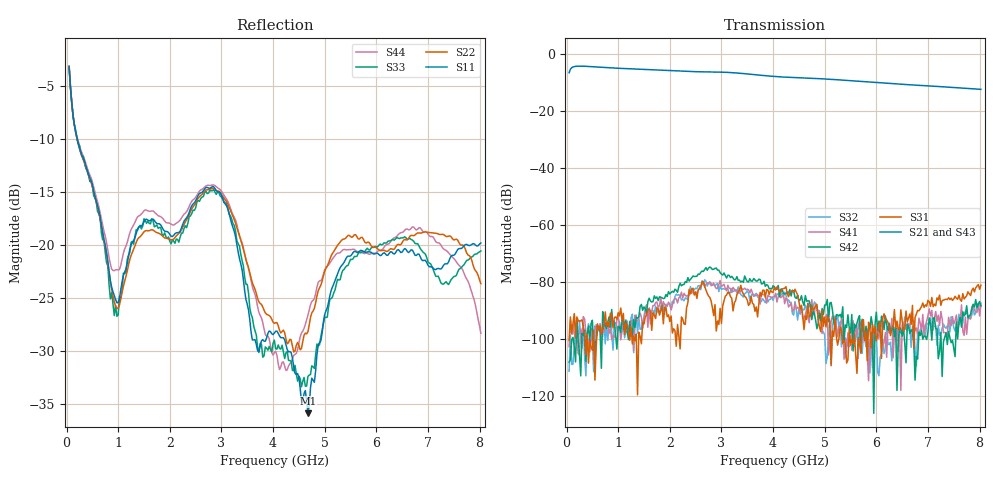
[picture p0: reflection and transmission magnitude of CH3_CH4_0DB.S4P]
!Agilent Technologies,E5071C,MY46316741,A.11.02
!Date: Thu May 28 15:05:39 2026
!Data & Calibration Information:
!1:CH3 INPUT 2:CH3 OUTPUT 3:CH4 INPUT 4:CH4 OUTPUT
!Freq	S11:SOLT4(ON)	S12:SOLT4(ON)	S13:SOLT4(ON)	S14:SOLT4(ON)
!	S21:SOLT4(ON)	S22:SOLT4(ON)	S23:SOLT4(ON)	S24:SOLT4(ON)
!	S31:SOLT4(ON)	S32:SOLT4(ON)	S33:SOLT4(ON)	S34:SOLT4(ON)
!	S41:SOLT4(ON)	S42:SOLT4(ON)	S43:SOLT4(ON)	S44:SOLT4(ON)
!PortZ  Port1:50+j0  Port2:50+j0  Port3:50+j0  Port4:50+j0
!Above PortZ is port z conversion or system Z0 setting when saving the data.
!When reading, reference impedance value at option line is always used.
# Hz S dB R 50
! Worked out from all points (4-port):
!   320 points, 50 MHz to 8.025 GHz, reference 50 ohm
!   strongest paths, dB at 50 MHz, 2.05 GHz, 4.05 GHz, 6.05 GHz, 8.025 GHz:
!     S21: -6.5, -5.8, -7.8, -10.0, -12.3
!     S43: -6.5, -5.8, -7.9, -10.1, -12.5
!     S31: -100.5, -97.9, -82.8, -95.1, -81.1
!     S42: -108.2, -83.3, -82.6, -93.7, -88.4
!     S41: -102.7, -88.1, -84.0, -99.9, -88.1
!     S32: -111.4, -86.8, -85.2, -113.0, -87.4
!   lowest |S11| = -35.9 dB at 4.675 GHz (marker M1), VSWR 1.03, Z = 49 - j1.26 ohm
!   |S11| at or under -10 dB: 206 MHz to end of sweep
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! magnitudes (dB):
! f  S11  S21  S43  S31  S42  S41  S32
! 50 MHz  -3.2  -6.5  -6.5  -100.5  -108.2  -102.7  -111.4
! 925 MHz  -24.8  -4.9  -4.9  -92.5  -93.7  -99.4  -94.5
! 2.85 GHz  -14.5  -6.3  -6.3  -91.8  -75.5  -80.4  -80.9
! 4.125 GHz  -28.6  -7.9  -8.0  -83.2  -85.2  -83.9  -84.9
! 4.675 GHz  -35.9  -8.4  -8.5  -87.5  -86.6  -92.2  -87.5
! 5.425 GHz  -21.2  -9.2  -9.2  -108.5  -96.0  -103.0  -100.2
! 8.025 GHz  -19.8  -12.3  -12.5  -81.1  -88.4  -88.1  -87.4
